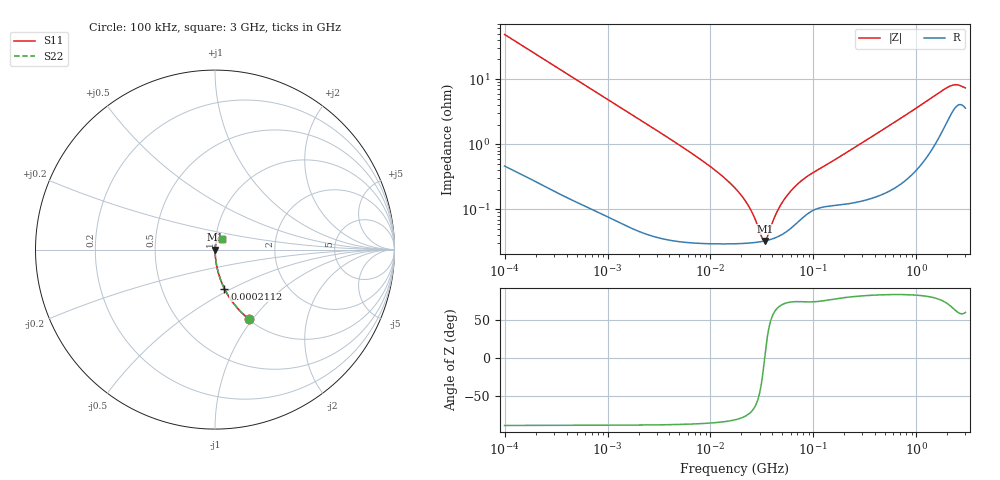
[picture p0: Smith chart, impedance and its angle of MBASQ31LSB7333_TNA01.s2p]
! MBASQ31LSB7333_TNA01  S-PARAMETER MODEL  ( Standard Model )
! Model Generated by TAIYO YUDEN Corporation (http://www.ty-top.com)
! Version 2.0
! TAIYO YUDEN Control No. 220822
! Copyright(c) 2013 TAIYO YUDEN CO.,LTD. All Rights Reserved.
! Product Description (link to TY-COMPAS)
! https://ds.yuden.co.jp/TYCOMPAS/or/detail?pn=MBASQ31LSB7333KTNA01&u=M
! Products Name : Multilayer Ceramic Capacitors
! Characteristics :
!  Capacitance : 0.033 [uF] , Rated Voltage : 250 [V] , TCC : X7R
!  Case Size : 3.2 x 1.6 / 0.126 x 0.063 [mm/inch] , Thickness : 1.6 / 0.063 [mm/inch]
!  (Conditions: Temperature = 25 [degC] , DC Bias Voltage = 0 [V])
! External Node Assignments :
!  1  o---| |---o  2
! GND o---------o GND
! Frequency Range : 100kHz  -  3GHz  [ 401 STEP ]
# MHZ S RI R 50
! Freq[MHz].  S11 Real  S11 Imag  S21 Real  S21 Imag  S12 Real  S12 Imag  S22 Real  S22 Imag
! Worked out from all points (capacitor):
!   401 points, 100 kHz to 3 GHz, reference 50 ohm
!   read as one part in series: C = 32.8 nF near 105.3 kHz
!   lowest |Z| = 33 mohm at 33.85 MHz (marker M1)
!   series resonance near 33.62 MHz, so ESL is about 680 pH
!   S11 on the Smith chart (normalised r, x): 100 kHz: 1.01, -0.97; 211.2 kHz: 1.01, -0.46; 3 GHz: 1.07, +0.13
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0.1  0.192 -0.3891  0.808 0.3891  0.808 0.3891  0.192 -0.3891
0.14345  0.105 -0.3014  0.895 0.3014  0.895 0.3014  0.105 -0.3014
0.21115  0.0525 -0.2175  0.9475 0.2175  0.9475 0.2175  0.0525 -0.2175
0.562235  0.00867 -0.0861  0.9913 0.0861  0.9913 0.0861  0.00867 -0.0861
3.161081  0.000605 -0.0155  0.9994 0.0155  0.9994 0.0155  0.000605 -0.0155
9.824692  0.000318 -0.00461  0.9997 0.00461  0.9997 0.00461  0.000318 -0.00461
13.7349  0.000304 -0.00301  0.9997 0.00301  0.9997 0.00301  0.000304 -0.00301
17.7727  0.000301 -0.00201  0.9997 0.00201  0.9997 0.00201  0.000301 -0.00201
23.59795  0.000305 -0.00107  0.9997 0.00107  0.9997 0.00107  0.000305 -0.00107
26.84345  0.000311 -0.000674  0.9997 0.000674  0.9997 0.000674  0.000311 -0.000674
31.3325  0.000321 -0.000209  0.9997 0.000209  0.9997 0.000209  0.000321 -0.000209
32.98988  0.000326 -5.58e-05  0.9997 5.58e-05  0.9997 5.58e-05  0.000326 -5.58e-05
33.85116  0.000329 2.1e-05  0.9997 -2.1e-05  0.9997 -2.1e-05  0.000329 2.1e-05
35.64176  0.000335 0.000175  0.9997 -0.000175  0.9997 -0.000175  0.000335 0.000175
44.94634  0.000381 0.000882  0.9996 -0.000882  0.9996 -0.000882  0.000381 0.000882
53.83243  0.000449 0.00146  0.9996 -0.00146  0.9996 -0.00146  0.000449 0.00146
69.65816  0.00063 0.00233  0.9994 -0.00233  0.9994 -0.00233  0.00063 0.00233
97.38194  0.000959 0.00347  0.999 -0.00347  0.999 -0.00347  0.000959 0.00347
547.5153  0.00227 0.0192  0.9977 -0.0192  0.9977 -0.0192  0.00227 0.0192
2038.117  0.028 0.068  0.972 -0.068  0.972 -0.068  0.028 0.068
2441.062  0.0411 0.0672  0.9589 -0.0672  0.9589 -0.0672  0.0411 0.0672
3000  0.0382 0.0592  0.9618 -0.0592  0.9618 -0.0592  0.0382 0.0592
